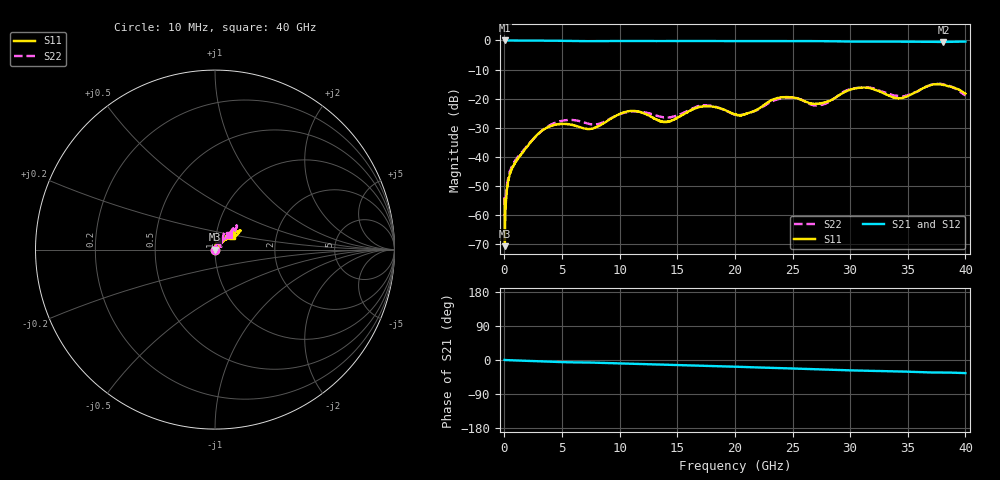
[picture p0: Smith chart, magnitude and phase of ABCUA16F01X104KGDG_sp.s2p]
! Amotech Co.,Ltd.
! http://www.amotech.co.kr/
! Date: Wednesday, December 02, 2020 17:28:45
! Part Number: ABCUA 16F 01X 104K GDG
! Freq. Start=10[MHz] Stop=40[GHz], 4000[Steps]
# Hz S  dB  R 50
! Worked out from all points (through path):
!   4000 points, 10 MHz to 40 GHz, reference 50 ohm
!   highest |S21| = 0.00 dB at 30 MHz (marker M1); lowest = -0.5 dB at 38.09 GHz (marker M2)
!   group delay of S21, straight-line fit = 2.42 ps
!   lowest |S11| = -70.7 dB at 30 MHz (marker M3), VSWR 1.00, Z = 50 - j0.0114 ohm
!   |S11| at or under -10 dB: start of sweep to end of sweep
!   |S22| runs from -60.4 to -14.9 dB; largest |S21 - S12| = 0.0034
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1e7  -54.47 -94.8  -0.00 0.1  0.00 0.2  -53.81 -63.6
3e7  -70.69 -157.0  -0.00 -0.0  0.00 -0.0  -60.37 -7.9
2.2e8  -51.01 75.8  -0.01 -0.3  -0.01 -0.3  -49.57 57.7
4e8  -46.96 69.1  -0.02 -0.5  -0.02 -0.5  -46.02 59.5
6.8e8  -43.86 67.6  -0.03 -0.8  -0.03 -0.8  -43.02 60.8
2.87e9  -32.30 84.1  -0.05 -3.1  -0.04 -3.0  -32.35 72.6
4.62e9  -28.79 73.3  -0.12 -5.1  -0.11 -5.1  -27.96 61.0
6.68e9  -29.97 36.1  -0.26 -6.4  -0.25 -6.4  -27.92 25.7
8.08e9  -29.60 37.6  -0.22 -7.2  -0.21 -7.2  -28.76 35.4
1.089e10  -24.23 58.9  -0.20 -9.8  -0.20 -9.7  -24.49 59.3
1.334e10  -27.42 53.9  -0.21 -11.8  -0.20 -11.8  -25.99 44.4
1.437e10  -27.73 52.4  -0.21 -12.7  -0.20 -12.6  -26.43 40.5
1.725e10  -22.67 55.9  -0.20 -15.3  -0.20 -15.2  -22.26 58.1
2.001e10  -25.49 49.8  -0.19 -17.6  -0.18 -17.6  -25.48 51.8
2.399e10  -19.56 49.5  -0.22 -21.6  -0.22 -21.4  -19.95 61.1
2.667e10  -21.73 44.9  -0.23 -24.0  -0.22 -23.8  -22.06 54.0
3.079e10  -16.28 46.8  -0.42 -27.7  -0.41 -27.6  -16.29 49.4
3.334e10  -18.88 44.7  -0.40 -29.7  -0.39 -29.6  -18.20 44.2
3.464e10  -19.61 36.5  -0.41 -30.5  -0.40 -30.4  -19.11 39.9
3.691e10  -15.46 36.1  -0.47 -32.8  -0.46 -32.7  -15.42 45.1
3.809e10  -15.29 37.7  -0.51 -33.1  -0.50 -33.0  -15.05 47.9
4e10  -18.31 38.2  -0.39 -34.5  -0.38 -34.4  -18.96 47.8
